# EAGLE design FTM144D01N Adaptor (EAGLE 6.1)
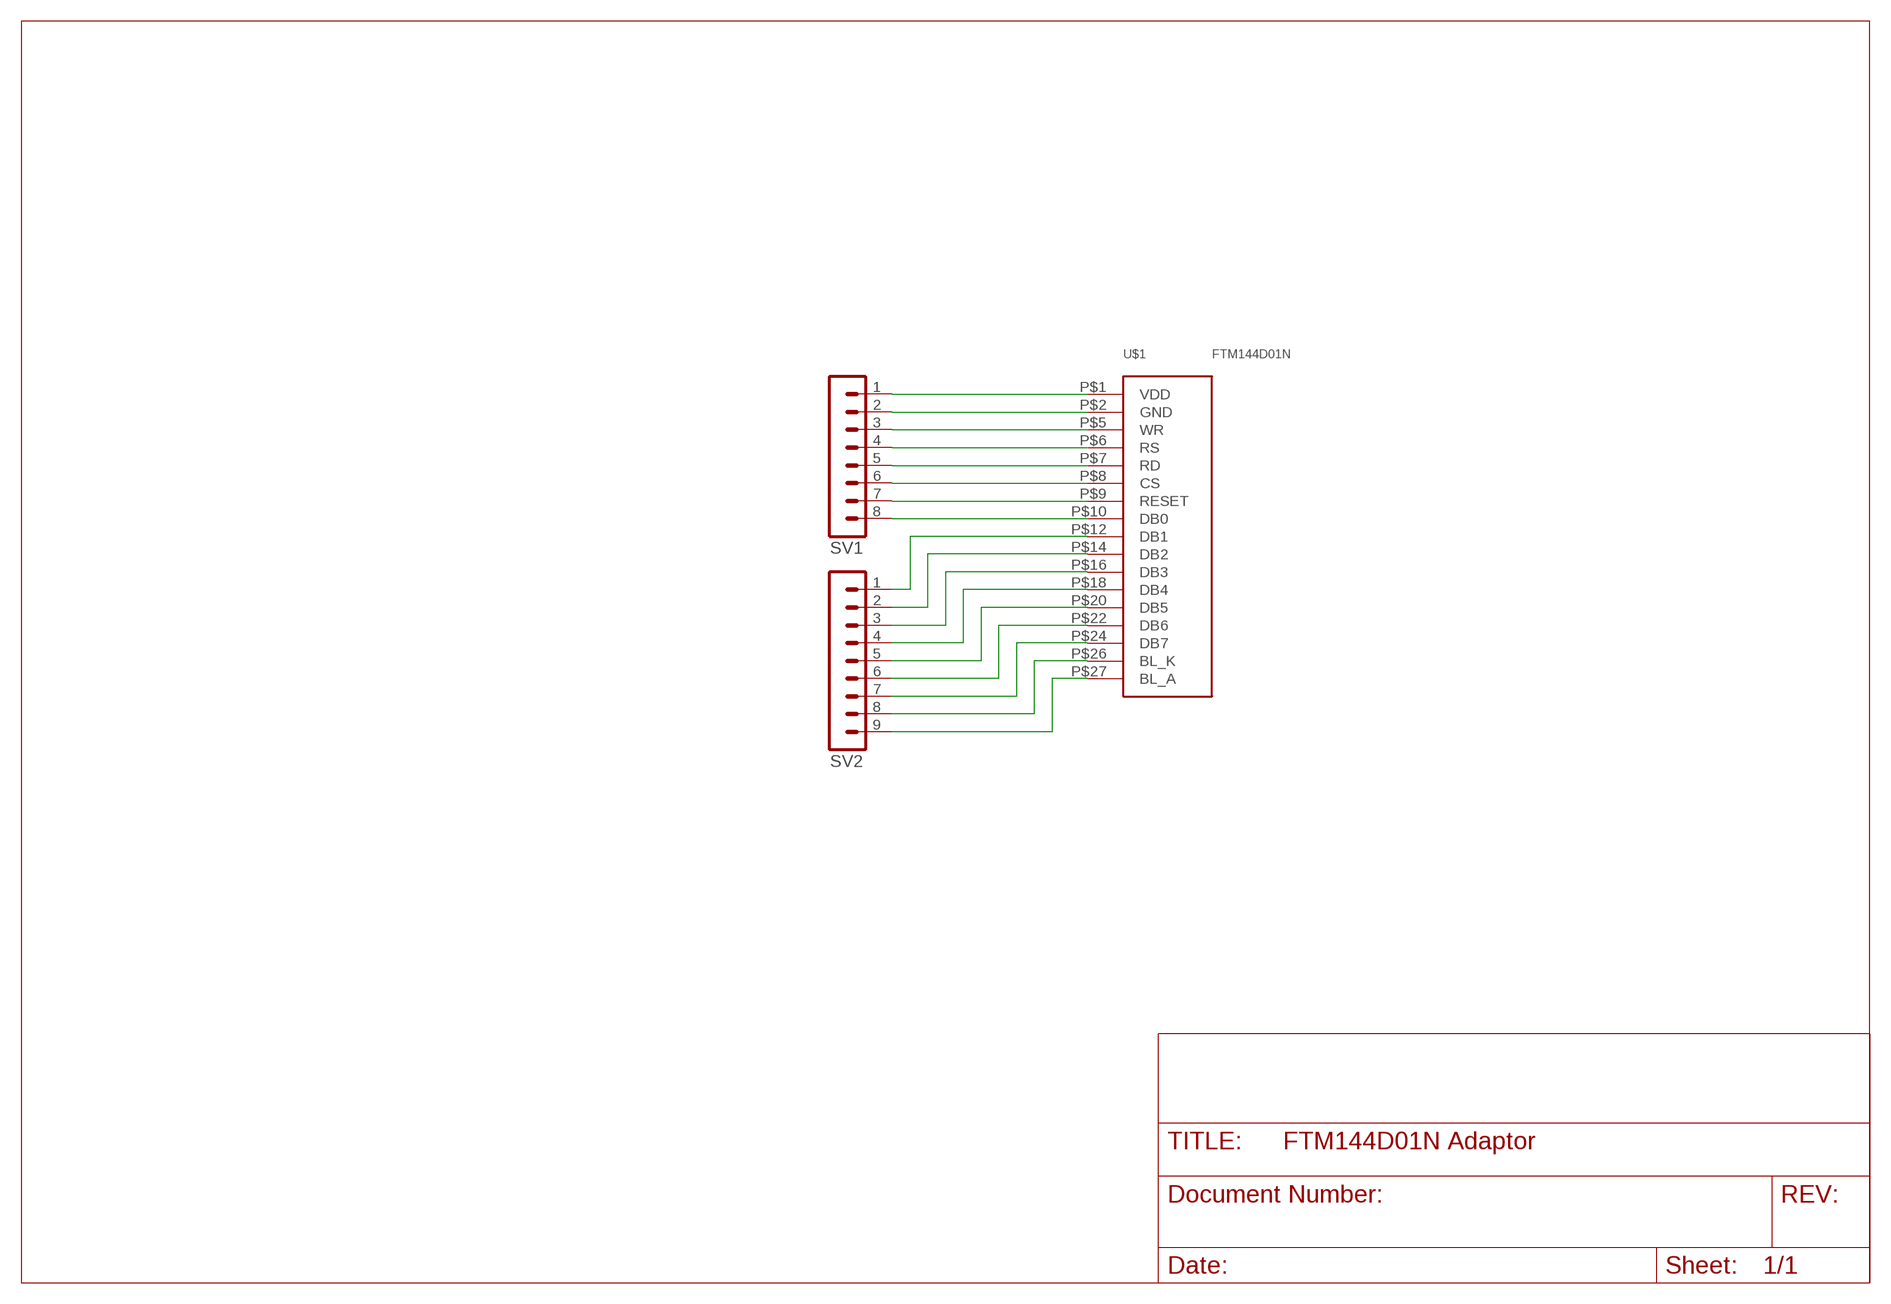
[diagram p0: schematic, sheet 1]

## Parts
SV1  MA08-1  [MA08-1]
SV2  MA09-1  [MA09-1]
U$1  FTM144D01N  [FTM144D01N]

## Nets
N$1: SV1.1 U$1.P$1(VDD)
N$2: SV1.2 U$1.P$2(GND)
N$3: SV1.3 U$1.P$5(WR)
N$4: SV1.4 U$1.P$6(RS)
N$5: SV1.5 U$1.P$7(RD)
N$6: SV1.6 U$1.P$8(CS)
N$7: SV1.7 U$1.P$9(RESET)
N$8: SV1.8 U$1.P$10(DB0)
N$9: SV2.1 U$1.P$12(DB1)
N$10: SV2.2 U$1.P$14(DB2)
N$11: SV2.3 U$1.P$16(DB3)
N$12: SV2.4 U$1.P$18(DB4)
N$13: SV2.5 U$1.P$20(DB5)
N$14: SV2.6 U$1.P$22(DB6)
N$15: SV2.7 U$1.P$24(DB7)
N$16: SV2.8 U$1.P$26(BL_K)
N$17: SV2.9 U$1.P$27(BL_A)

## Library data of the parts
SV1 = con-lstb:MA08-1: PIN HEADER; OC_FARNELL: unknown; OC_NEWARK: unknown
SV2 = con-lstb:MA09-1: PIN HEADER; OC_FARNELL: unknown; OC_NEWARK: unknown
U$1 = simonslbr:FTM144D01N: FTM144D01N TFT LCD 128x128 65K colour TFT LCD with ILITEK ILI9163 driver IC 0.8mm pitch 'hot-bar' solder connector

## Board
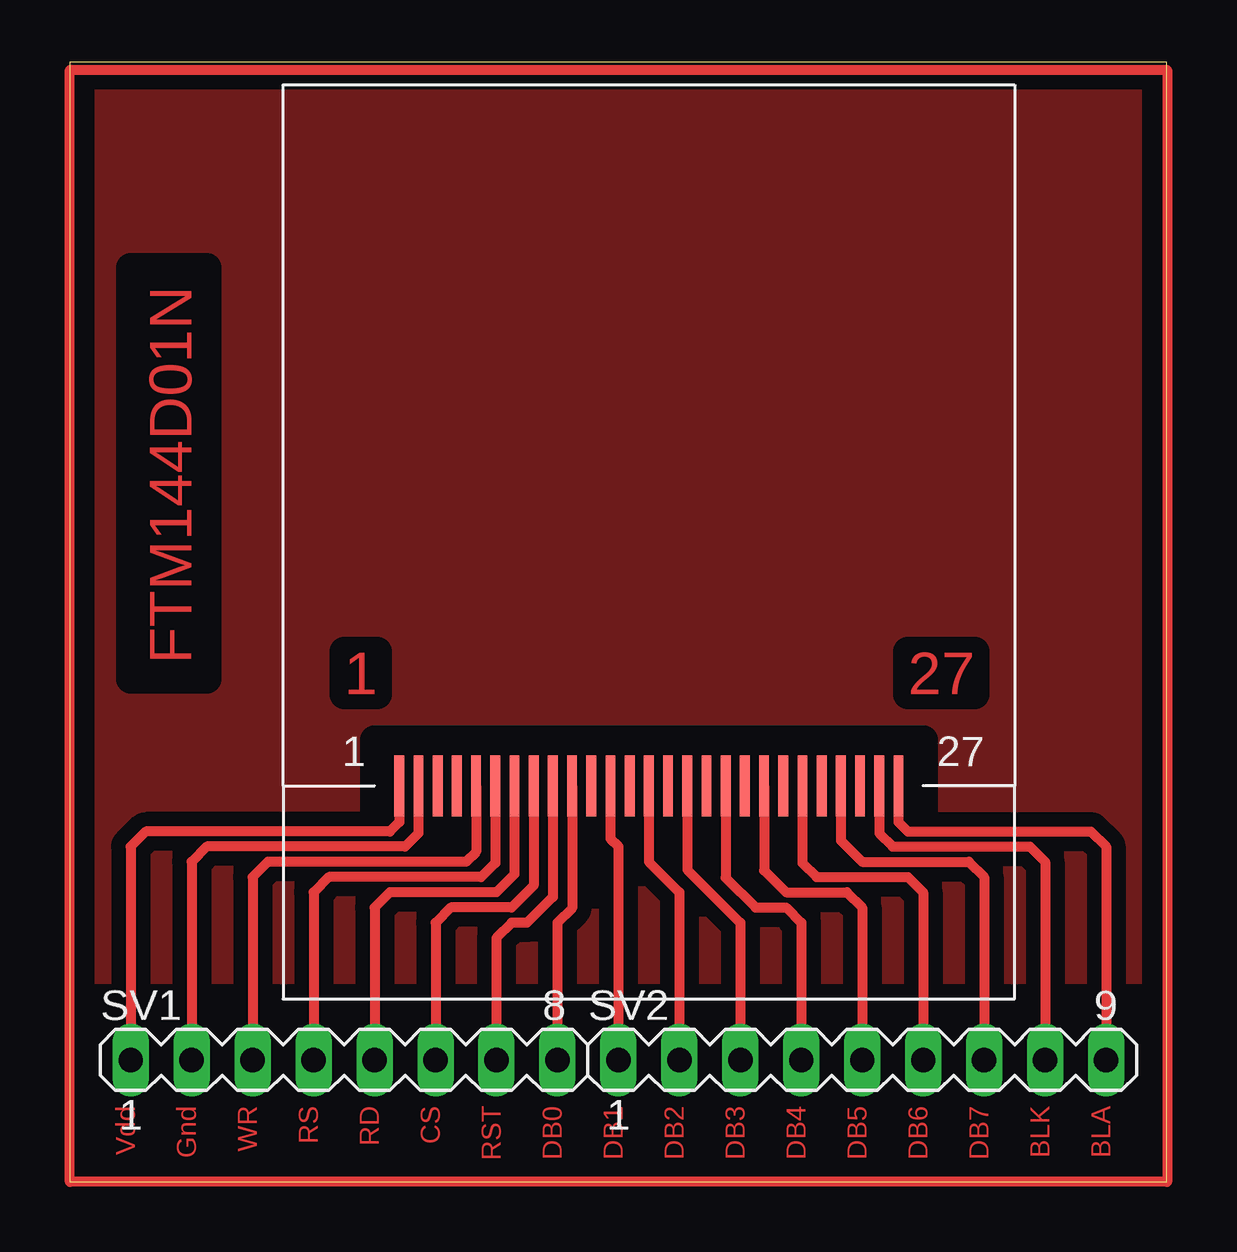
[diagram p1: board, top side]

Size 45.7 x 46.66 mm. Coordinates in mm from the lower left corner, seen from the top.
Outline: 0,0 45.7,0 45.7,46.66 0,46.66 0,0
Copper layers (1*16): Top 0.035mm / dielectric 1.5mm / Bottom 0.035mm
Design rules: minimum track width 10mil, minimum drill 24mil, track to track 8mil, track to pad 8mil, pad to pad 8mil, via to via 8mil, smd to smd 8mil, copper to edge 40mil, drill to drill 8mil, minimum pad ring 10mil, minimum via ring 8mil, stop-mask expansion 4mil, vias tented up to drill 0mil, thermal gap 10mil
tRestrict: area 1.3,0.6 to 44.5,7.6; area 12.7,14 to 35.6,18.4; area 2.5,21 to 5.7,38.1

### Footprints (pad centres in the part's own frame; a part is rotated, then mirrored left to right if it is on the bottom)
MA08-1 = drill 1.016 long: 1 -8.89,0; 2 -6.35,0; 3 -3.81,0; 4 -1.27,0; 5 1.27,0; 6 3.81,0; 7 6.35,0; 8 8.89,0
MA09-1 = drill 1.016 long: 1 -10.16,0; 2 -7.62,0; 3 -5.08,0; 4 -2.54,0; 5 0,0; 6 2.54,0; 7 5.08,0; 8 7.62,0; 9 10.16,0
FTM144D01N = smd 0.406 x 2.54: P$1 -10.4,0; P$2 -9.6,0; P$3 -8.8,0; P$4 -8,0; P$5 -7.2,0; P$6 -6.4,0; P$7 -5.6,0; P$8 -4.8,0; P$9 -4,0; P$10 -3.2,0; P$11 -2.4,0; P$12 -1.6,0; P$13 -0.8,0; P$14 0,0; P$15 0.8,0; P$16 1.6,0; P$17 2.4,0; P$18 3.2,0; P$19 4,0; P$20 4.8,0; P$21 5.6,0; P$22 6.4,0; P$23 7.2,0; P$24 8,0; P$25 8.8,0; P$26 9.6,0; P$27 10.4,0

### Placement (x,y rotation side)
SV1  11.43,5.08 0 top
SV2  33.02,5.08 0 top
U$1  24.13,16.51 0 top

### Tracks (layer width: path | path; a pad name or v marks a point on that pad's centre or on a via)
N$1
  Top 0.406: U$1.P$1 13.73,15 13.34,14.61 3.17,14.61 2.54,13.97 SV1.1
N$2
  Top 0.406: U$1.P$2 14.53,14.53 13.97,13.97 5.71,13.97 5.08,13.34 SV1.2
N$3
  Top 0.406: U$1.P$5 16.93,13.76 16.51,13.34 8.26,13.34 7.62,12.7 SV1.3
N$4
  Top 0.406: U$1.P$6 17.73,13.29 17.14,12.7 10.79,12.7 10.16,12.06 SV1.4
N$5
  Top 0.406: U$1.P$7 18.53,12.81 17.78,12.06 13.34,12.06 12.7,11.43 SV1.5
N$6
  Top 0.406: U$1.P$8 19.33,12.35 18.41,11.43 15.88,11.43 15.24,10.79 SV1.6
N$7
  Top 0.406: U$1.P$9 20.13,11.88 19.05,10.79 18.41,10.79 17.78,10.16 SV1.7
N$8
  Top 0.406: U$1.P$10 20.93,11.4 20.32,10.79 SV1.8
N$9
  Top 0.406: U$1.P$12 22.53,14.3 22.86,13.97 SV2.1
N$10
  Top 0.406: U$1.P$14 24.13,13.34 25.4,12.06 SV2.2
N$11
  Top 0.406: U$1.P$16 25.73,13.01 27.94,10.79 SV2.3
N$12
  Top 0.406: U$1.P$18 27.33,12.68 28.57,11.43 29.84,11.43 30.48,10.79 SV2.4
N$13
  Top 0.406: U$1.P$20 28.93,12.98 29.84,12.06 32.38,12.06 33.02,11.43 SV2.5
N$14
  Top 0.406: U$1.P$22 30.53,13.29 31.11,12.7 34.92,12.7 35.56,12.06 SV2.6
N$15
  Top 0.406: U$1.P$24 32.13,14.22 33.02,13.34 37.47,13.34 38.1,12.7 SV2.7
N$16
  Top 0.406: U$1.P$26 33.73,14.53 34.29,13.97 40.01,13.97 40.64,13.34 SV2.8
N$17
  Top 0.406: U$1.P$27 34.53,15 34.92,14.61 42.55,14.61 43.18,13.97 SV2.9
N$18
  Top 0.406: 0,46.35 45.72,46.35 45.72,0 0,0 0,46.35
N$19
  pour Top (isolate 0.61): 0,46.35 45.72,46.35 45.72,0 0,0

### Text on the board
Top: FTM144D01N | 1 | 27 | Vdd | Gnd | WR | RS | RD | CS | RST | DB0 | DB1 | DB2 | DB3 | DB4 | DB5 | DB6 | DB7 | BLK | BLA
